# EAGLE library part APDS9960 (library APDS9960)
APDS9960 手势传感器
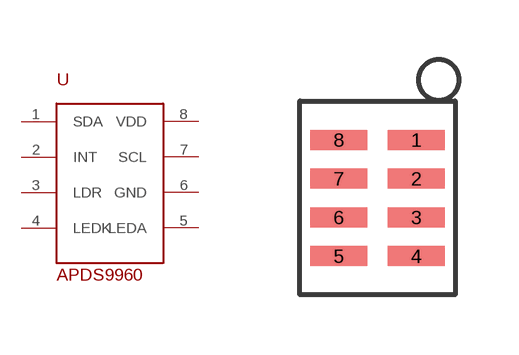
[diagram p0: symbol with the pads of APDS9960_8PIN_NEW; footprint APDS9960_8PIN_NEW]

Designator prefix U

## APDS9960  [APDS9960_8PIN_NEW]
1  SDA
2  INT
3  LDR
4  LEDK
5  LEDA
6  GND
7  SCL
8  VDD

## Footprint APDS9960_8PIN_NEW (pad centres in mm)
smd 1.422 x 0.5: 1 1.94,0; 2 1.94,-0.97; 3 1.94,-1.94; 4 1.94,-2.91; 5 0,-2.91; 6 0,-1.94; 7 0,-0.97; 8 0,0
